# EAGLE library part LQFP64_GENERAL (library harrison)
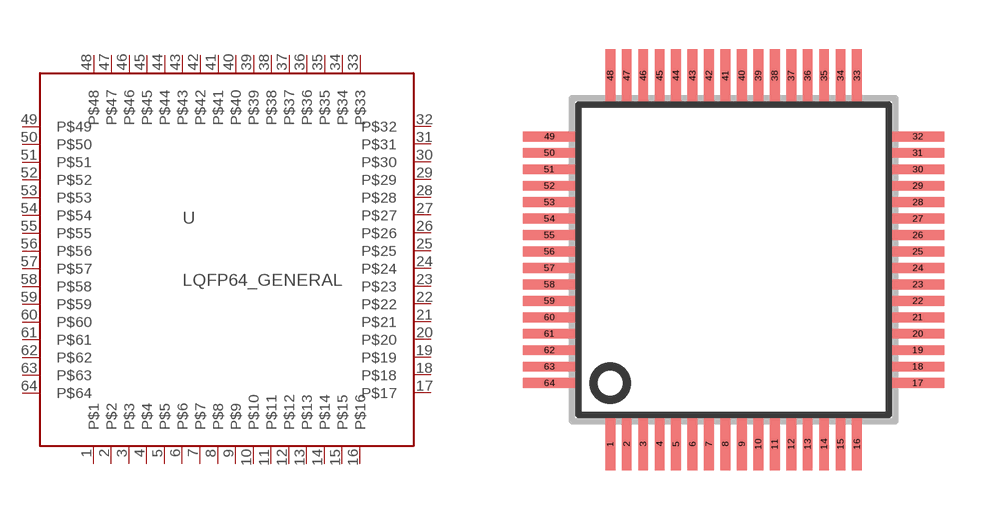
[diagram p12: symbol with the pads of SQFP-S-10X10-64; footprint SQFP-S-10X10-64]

Designator prefix -

## LQFP64_GENERAL  [SQFP-S-10X10-64]
1  P$1
2  P$2
3  P$3
4  P$4
5  P$5
6  P$6
7  P$7
8  P$8
9  P$9
10  P$10
11  P$11
12  P$12
13  P$13
14  P$14
15  P$15
16  P$16
17  P$17
18  P$18
19  P$19
20  P$20
21  P$21
22  P$22
23  P$23
24  P$24
25  P$25
26  P$26
27  P$27
28  P$28
29  P$29
30  P$30
31  P$31
32  P$32
33  P$33
34  P$34
35  P$35
36  P$36
37  P$37
38  P$38
39  P$39
40  P$40
41  P$41
42  P$42
43  P$43
44  P$44
45  P$45
46  P$46
47  P$47
48  P$48
49  P$49
50  P$50
51  P$51
52  P$52
53  P$53
54  P$54
55  P$55
56  P$56
57  P$57
58  P$58
59  P$59
60  P$60
61  P$61
62  P$62
63  P$63
64  P$64

## Footprint SQFP-S-10X10-64 (pad centres in mm)
smd 0.3 x 1.6: 1 -3.75,-5.6; 2 -3.25,-5.6; 3 -2.75,-5.6; 4 -2.25,-5.6; 5 -1.75,-5.6; 6 -1.25,-5.6; 7 -0.75,-5.6; 8 -0.25,-5.6; 9 0.25,-5.6; 10 0.75,-5.6; 11 1.25,-5.6; 12 1.75,-5.6; 13 2.25,-5.6; 14 2.75,-5.6; 15 3.25,-5.6; 16 3.75,-5.6; 33 3.75,5.6; 34 3.25,5.6; 35 2.75,5.6; 36 2.25,5.6; 37 1.75,5.6; 38 1.25,5.6; 39 0.75,5.6; 40 0.25,5.6; 41 -0.25,5.6; 42 -0.75,5.6; 43 -1.25,5.6; 44 -1.75,5.6; 45 -2.25,5.6; 46 -2.75,5.6; 47 -3.25,5.6; 48 -3.75,5.6
smd 1.6 x 0.3: 17 5.6,-3.75; 18 5.6,-3.25; 19 5.6,-2.75; 20 5.6,-2.25; 21 5.6,-1.75; 22 5.6,-1.25; 23 5.6,-0.75; 24 5.6,-0.25; 25 5.6,0.25; 26 5.6,0.75; 27 5.6,1.25; 28 5.6,1.75; 29 5.6,2.25; 30 5.6,2.75; 31 5.6,3.25; 32 5.6,3.75; 49 -5.6,3.75; 50 -5.6,3.25; 51 -5.6,2.75; 52 -5.6,2.25; 53 -5.6,1.75; 54 -5.6,1.25; 55 -5.6,0.75; 56 -5.6,0.25; 57 -5.6,-0.25; 58 -5.6,-0.75; 59 -5.6,-1.25; 60 -5.6,-1.75; 61 -5.6,-2.25; 62 -5.6,-2.75; 63 -5.6,-3.25; 64 -5.6,-3.75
